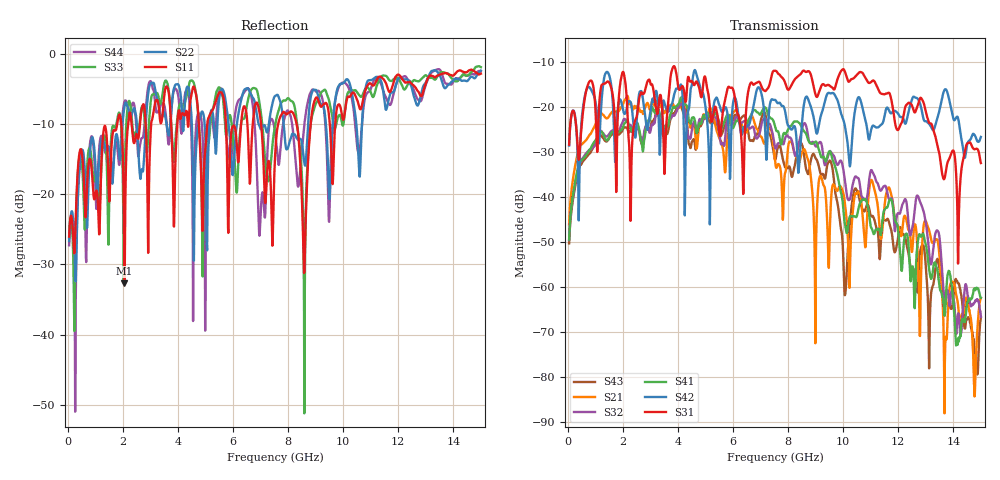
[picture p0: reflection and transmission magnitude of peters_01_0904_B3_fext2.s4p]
# MHZ S RI R 50.00
! FREQ  S11  S12  S13  S14
!  S21  S22  S23  S24
!  S31  S32  S33  S34
!  S41  S42  S43  S44
!  REAL  IMAG  REAL  IMAG  REAL  IMAG  REAL  IMAG
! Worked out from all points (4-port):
!   1496 points, 50 MHz to 15 GHz, reference 50 ohm
!   strongest paths, dB at 50 MHz, 3.79 GHz, 7.53 GHz, 11.27 GHz, 15 GHz:
!     S31: -28.3, -11.6, -11.9, -15.9, -32.4
!     S42: -28.5, -19.2, -18.4, -24.5, -26.6
!     S41: -49.5, -20.5, -24.3, -47.1, -62.4
!     S32: -49.5, -21.9, -29.0, -37.2, -66.7
!     S21: -46.1, -19.4, -32.2, -42.7, -62.5
!     S43: -50.3, -21.7, -31.7, -48.3, -66.8
!   lowest |S11| = -32.7 dB at 2.06 GHz (marker M1), VSWR 1.05, Z = 47.7 + j0.165 ohm
!   |S11| at or under -10 dB: start of sweep to 1.793 GHz; 5.742 GHz to 6.293 GHz (550.2 MHz wide, 9.14 % of centre); 7.021 GHz to 7.638 GHz (617.2 MHz wide, 8.42 % of centre)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
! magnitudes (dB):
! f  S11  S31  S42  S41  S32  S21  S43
! 50 MHz  -26.0  -28.3  -28.5  -49.5  -49.5  -46.1  -50.3
! 2.06 GHz  -32.7  -13.2  -21.5  -23.6  -22.6  -18.4  -24.5
! 2.28 GHz  -8.6  -45.3  -18.8  -24.5  -23.9  -18.9  -25.2
! 8.02 GHz  -8.4  -16.1  -24.2  -24.7  -26.7  -28.1  -33.3
! 8.6 GHz  -29.9  -11.9  -18.6  -25.5  -23.5  -29.4  -31.7
! 9.25 GHz  -7.3  -14.9  -20.8  -31.1  -29.5  -36.6  -34.8
! 15 GHz  -2.8  -32.4  -26.6  -62.4  -66.7  -62.5  -66.8
